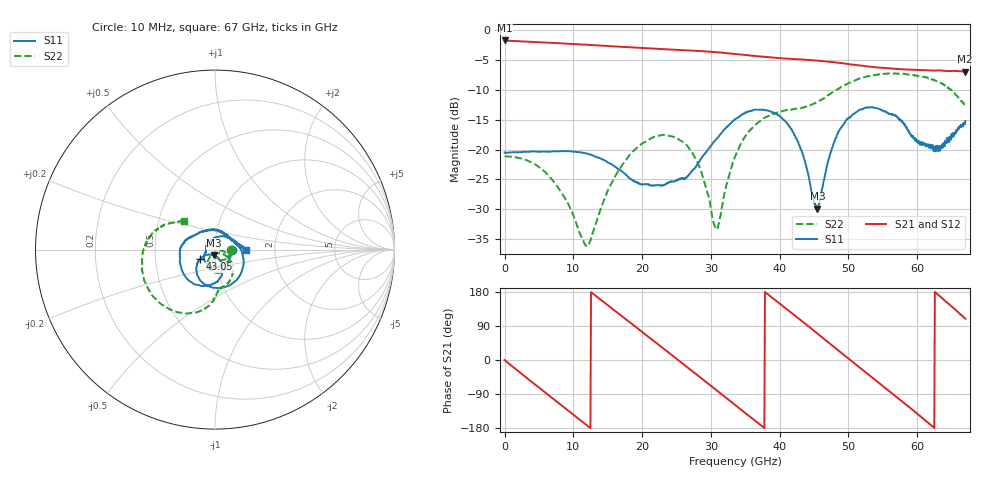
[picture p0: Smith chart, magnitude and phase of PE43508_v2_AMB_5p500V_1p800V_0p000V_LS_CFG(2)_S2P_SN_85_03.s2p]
!Keysight Technologies,N5227A,US51270237,A.10.43.00
!Date: Wednesday, August 22, 2018 17:06:42
!Correction: S11(Full 2 Port(1,3))
!S31(Full 2 Port(1,3))
!S13(Full 2 Port(1,3))
!S33(Full 2 Port(1,3))
!S2P File: Measurements: S11, S31, S13, S33:
# Hz S  dB  R 50
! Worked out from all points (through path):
!   801 points, 10 MHz to 67 GHz, reference 50 ohm
!   highest |S21| = -1.77 dB at 10 MHz (marker M1); lowest = -7.0 dB at 66.92 GHz (marker M2)
!   group delay of S21, straight-line fit = 39.9 ps
!   lowest |S11| = -29.9 dB at 45.48 GHz (marker M3), VSWR 1.07, Z = 49.5 - j3.14 ohm
!   |S11| at or under -10 dB: start of sweep to end of sweep
!   |S22| runs from -36.1 to -7.2 dB; largest |S21 - S12| = 0.0052
!   S11 on the Smith chart (normalised r, x): 10 MHz: 1.21, -0.00; 43.05 GHz: 0.84, -0.09; 67 GHz: 1.42, -0.01
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1e7  -20.49 -0.5  -1.77 -0.2  -1.77 -0.2  -21.12 -0.8
2.522125e9  -20.42 -28.2  -1.92 -37.2  -1.92 -37.2  -21.52 -29.5
5.70415e9  -20.33 -60.5  -2.10 -83.0  -2.10 -83.0  -23.56 -62.7
8.216275e9  -20.28 -84.9  -2.26 -118.9  -2.25 -118.9  -27.12 -83.2
1.123082e10  -20.49 -111.4  -2.44 -161.9  -2.44 -161.8  -34.67 -73.0
1.223568e10  -20.76 -120.4  -2.51 -176.1  -2.51 -176.1  -35.81 -39.6
1.40779e10  -21.57 -135.6  -2.63 157.8  -2.63 157.8  -29.62 -9.8
1.734366e10  -23.88 -156.8  -2.86 111.6  -2.85 111.6  -22.21 -23.4
1.977205e10  -25.82 -166.3  -3.02 77.3  -3.01 77.3  -19.17 -44.2
2.236791e10  -25.95 -178.2  -3.19 40.7  -3.18 40.7  -17.72 -69.5
2.630358e10  -24.84 117.2  -3.41 -15.1  -3.41 -15.2  -19.03 -107.7
3.074166e10  -18.33 19.3  -3.73 -78.9  -3.73 -78.8  -33.30 -85.2
3.3505e10  -14.99 -27.3  -4.01 -118.7  -4.01 -118.6  -21.22 -31.8
3.802682e10  -13.43 -90.5  -4.53 177.0  -4.53 177.1  -14.55 -61.7
4.305108e10  -19.96 -147.2  -4.94 105.4  -4.92 105.4  -13.11 -84.2
4.472582e10  -27.44 -140.6  -5.06 81.0  -5.05 81.0  -12.46 -86.8
4.547946e10  -29.90 -98.1  -5.14 69.9  -5.12 69.9  -12.00 -88.5
4.949886e10  -15.44 -83.2  -5.64 10.8  -5.64 10.8  -9.25 -102.1
5.586291e10  -14.07 -167.7  -6.42 -81.0  -6.42 -81.4  -7.28 -142.7
6.172454e10  -19.70 77.1  -6.77 -167.8  -6.80 -168.0  -8.07 178.3
6.691626e10  -15.80 1.2  -6.99 110.3  -7.04 110.5  -12.54 138.7
6.7e10  -15.22 -0.8  -6.98 108.9  -7.02 109.1  -12.62 137.1
